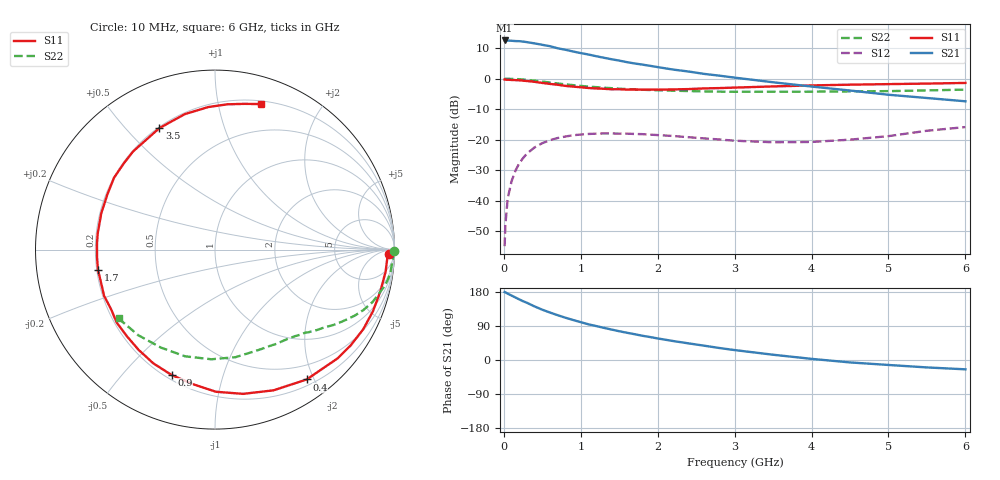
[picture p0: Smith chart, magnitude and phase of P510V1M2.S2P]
! SIEMENS Small Signal Semiconductors
! BFP183
! Si NPN RF Bipolar Junction Transistor in SOT143
! VCE = 10 V  IC = 1.2 mA
! Common Emitter S-Parameters:  March  1996
# GHz  S  MA  R  50
!  f  S11  S21  S12  S22
! GHz  MAG  ANG  MAG  ANG  MAG  ANG  MAG  ANG
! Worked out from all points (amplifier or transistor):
!   36 points, 10 MHz to 6 GHz, reference 50 ohm
!   highest |S21| = 12.5 dB at 10 MHz (marker M1)
!   |S21| within 3 dB of that: start of sweep to 790.3 MHz
!   unconditionally stable (mu >= 1): 2.46 GHz to end of sweep
!   at 250 MHz: K = 0.10, MSG = 19.1 dB, |S12| = -26.0 dB
!   at 1.4 GHz: K = 0.55, MSG = 12.1 dB, |S12| = -18.0 dB
!   at 6 GHz: K = 1.00, MAG = 3.9 dB, |S12| = -15.9 dB
!   S11 on the Smith chart (normalised r, x): 10 MHz: 41, -28; 400 MHz: 0.28, -1.90; 900 MHz: 0.22, -0.69; 1.7 GHz: 0.20, -0.08; 3.5 GHz: 0.21, +0.62; 6 GHz: 0.23, +1.34
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0.01  0.9675 -1.3  4.215 179.3  0.0018 85.8  0.9995 -0.5
0.02  0.9608 -2.9  4.195 178.6  0.004 84.0  0.9958 -1.1
0.05  0.9587 -7.3  4.194 175.0  0.0109 86.9  0.9939 -2.5
0.1  0.9502 -14.2  4.168 170.1  0.0208 80.7  0.9881 -5.0
0.15  0.9447 -21.4  4.117 165.0  0.0309 76.9  0.9855 -7.5
0.25  0.9255 -35.2  4.039 155.1  0.0499 69.0  0.9661 -12.2
0.4  0.8856 -54.8  3.774 141.3  0.0747 58.0  0.9253 -18.4
0.5  0.8493 -67.4  3.575 132.7  0.0876 50.9  0.8932 -22.1
0.6  0.8188 -79.0  3.394 125.2  0.0981 44.8  0.8622 -25.2
0.7  0.7921 -89.6  3.137 118.2  0.1064 39.3  0.8315 -27.9
0.8  0.7593 -99.6  2.968 111.6  0.1125 34.4  0.8053 -30.3
0.9  0.7392 -109.1  2.78 105.6  0.1181 30.0  0.7818 -32.5
1.1  0.7023 -127.3  2.482 94.2  0.1239 22.5  0.7397 -36.3
1.4  0.6676 -150.2  2.075 80.4  0.1265 13.5  0.697 -41.3
1.7  0.6619 -170.2  1.77 68.1  0.1239 7.0  0.6654 -45.9
1.9  0.6583 177.7  1.62 60.6  0.1208 4.0  0.6499 -48.8
2.2  0.665 162.4  1.406 50.1  0.1148 0.5  0.6335 -53.6
2.8  0.6993 136.6  1.118 31.7  0.1007 -0.9  0.6118 -64.5
3.5  0.7444 114.6  0.871 13.9  0.0906 5.5  0.6102 -79.2
4.5  0.7951 92.7  0.638 -6.4  0.1 20.7  0.6175 -105.6
5.5  0.8284 78.6  0.481 -19.6  0.1399 26.5  0.6407 -131.9
6  0.8495 72.6  0.425 -24.6  0.1607 23.9  0.6602 -144.5
